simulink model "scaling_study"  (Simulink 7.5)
settings: Solver=ode23t  StartTime=0.0  StopTime=6  RelTol=1e-6
undefined symbols (not defined in the file or in its folder): dfilt, DiscIntNeverNeededParam
libraries: powerlib x45, powerlib_extras x17, simulink x12, dsparch4 x2
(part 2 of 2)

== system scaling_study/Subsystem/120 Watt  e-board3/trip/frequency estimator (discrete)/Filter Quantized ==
  In : Inport
  Input Quantizer : DataTypeConversion  OutDataTypeMode=Specify via dialog  OutDataType=fixdt(1,16,15)  OutDataTypeStr=fixdt(1,16,15)  RndMeth=Round
  filter : dsparch4/Biquad Filter  DialogController=dspdialog.BiquadFilter  DialogControllerArgs=DataTag0  IIRFiltStruct=Direct form II  CoeffSource=Specify via dialog  BiQuadCoeffs=[1 -1.35890654546667 1 1 -1.77683423091592 0.868775728611993;1 1 0 1 -0.84680556917748 0]  a0Flag=Warning  IC=0  ICnum=0  ICden=0  firstCoeffMode=Binary point scaling  firstCoeffWordLength=16  firstCoeffFracLength=14  outputMode=Binary point scaling  outputWordLength=16  outputFracLength=11  accumMode=Binary point scaling  accumWordLength=40  accumFracLength=29  denAccumFracLength=29  prodOutputMode=Binary point scaling  prodOutputWordLength=32  prodOutputFracLength=29  denProdOutputFracLength=29  memoryMode=Binary point scaling  memoryWordLength=16  memoryFracLength=15  secondMemoryFracLength=15  roundingMode=Convergent  overflowMode=off  ScaleValues=[0.0483208011510974;0.227336456672284;1]  optimizeScaleValues=on  ScaleValueMode=Specify via input port (g)  scaleValueFracLength=17  stageInputMode=Binary point scaling  stageOutputMode=Binary point scaling  stageInputWordLength=16  stageInputFracLength=12  stageOutputWordLength=16  stageOutputFracLength=11  FilterSource=Specify via dialog  dfiltObjectName=dfilt.df2tsos([1 0.3 0.4],[1 0.1 0.2])
  Out : Outport
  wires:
  In/1 -> Input Quantizer/1
  Input Quantizer/1 -> filter/1
  filter/1 -> Out/1

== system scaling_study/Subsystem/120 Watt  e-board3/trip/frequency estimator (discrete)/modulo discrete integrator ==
  In1 : Inport
  Abs : Abs
  Constant1 : Constant  OutDataType=sfix(16)  OutScaling=2^0
  Discrete-Time Integrator : DiscreteIntegrator  ExternalReset=rising  InitialConditionSource=external  SampleTime=dt  OutDataType=fixdt(1, 16)  OutScaling=2^0  UpperSaturationLimit=100  LowerSaturationLimit=-100  ShowStatePort=on  ICPrevOutput=DiscIntNeverNeededParam  ICPrevScaledInput=DiscIntNeverNeededParam
  Gain1 : Gain  Gain=1+.0001  ParameterDataType=sfix(16)  ParameterScaling=2^0  OutDataType=sfix(16)  OutScaling=2^0
  IC : InitialCondition  Value=0
  Math Function : Math  Operator=rem  OutDataType=sfix(16)  OutScaling=2^0
  Relational Operator : RelationalOperator
  Out1 : Outport
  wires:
  Relational Operator/1 -> Discrete-Time Integrator/2
  Discrete-Time Integrator/State -> Gain1/1
  Gain1/1 -> Abs/1
  Constant1/1 -> Relational Operator/2, Math Function/2
  Abs/1 -> Relational Operator/1, Math Function/1
  In1/1 -> Discrete-Time Integrator/1
  Discrete-Time Integrator/1 -> Out1/1
  IC/1 -> Discrete-Time Integrator/3
  Math Function/1 -> IC/1

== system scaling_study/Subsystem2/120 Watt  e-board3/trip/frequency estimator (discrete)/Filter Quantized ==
  In : Inport
  Input Quantizer : DataTypeConversion  OutDataTypeMode=Specify via dialog  OutDataType=fixdt(1,16,15)  OutDataTypeStr=fixdt(1,16,15)  RndMeth=Round
  filter : dsparch4/Biquad Filter  DialogController=dspdialog.BiquadFilter  DialogControllerArgs=DataTag1  IIRFiltStruct=Direct form II  CoeffSource=Specify via dialog  BiQuadCoeffs=[1 -1.35890654546667 1 1 -1.77683423091592 0.868775728611993;1 1 0 1 -0.84680556917748 0]  a0Flag=Warning  IC=0  ICnum=0  ICden=0  firstCoeffMode=Binary point scaling  firstCoeffWordLength=16  firstCoeffFracLength=14  outputMode=Binary point scaling  outputWordLength=16  outputFracLength=11  accumMode=Binary point scaling  accumWordLength=40  accumFracLength=29  denAccumFracLength=29  prodOutputMode=Binary point scaling  prodOutputWordLength=32  prodOutputFracLength=29  denProdOutputFracLength=29  memoryMode=Binary point scaling  memoryWordLength=16  memoryFracLength=15  secondMemoryFracLength=15  roundingMode=Convergent  overflowMode=off  ScaleValues=[0.0483208011510974;0.227336456672284;1]  optimizeScaleValues=on  ScaleValueMode=Specify via input port (g)  scaleValueFracLength=17  stageInputMode=Binary point scaling  stageOutputMode=Binary point scaling  stageInputWordLength=16  stageInputFracLength=12  stageOutputWordLength=16  stageOutputFracLength=11  FilterSource=Specify via dialog  dfiltObjectName=dfilt.df2tsos([1 0.3 0.4],[1 0.1 0.2])
  Out : Outport
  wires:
  In/1 -> Input Quantizer/1
  Input Quantizer/1 -> filter/1
  filter/1 -> Out/1

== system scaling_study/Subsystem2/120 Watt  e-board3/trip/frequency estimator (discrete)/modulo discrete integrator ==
  In1 : Inport
  Abs : Abs
  Constant1 : Constant  OutDataType=sfix(16)  OutScaling=2^0
  Discrete-Time Integrator : DiscreteIntegrator  ExternalReset=rising  InitialConditionSource=external  SampleTime=dt  OutDataType=fixdt(1, 16)  OutScaling=2^0  UpperSaturationLimit=100  LowerSaturationLimit=-100  ShowStatePort=on  ICPrevOutput=DiscIntNeverNeededParam  ICPrevScaledInput=DiscIntNeverNeededParam
  Gain1 : Gain  Gain=1+.0001  ParameterDataType=sfix(16)  ParameterScaling=2^0  OutDataType=sfix(16)  OutScaling=2^0
  IC : InitialCondition  Value=0
  Math Function : Math  Operator=rem  OutDataType=sfix(16)  OutScaling=2^0
  Relational Operator : RelationalOperator
  Out1 : Outport
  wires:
  Relational Operator/1 -> Discrete-Time Integrator/2
  Discrete-Time Integrator/State -> Gain1/1
  Gain1/1 -> Abs/1
  Constant1/1 -> Relational Operator/2, Math Function/2
  Abs/1 -> Relational Operator/1, Math Function/1
  In1/1 -> Discrete-Time Integrator/1
  Discrete-Time Integrator/1 -> Out1/1
  IC/1 -> Discrete-Time Integrator/3
  Math Function/1 -> IC/1
